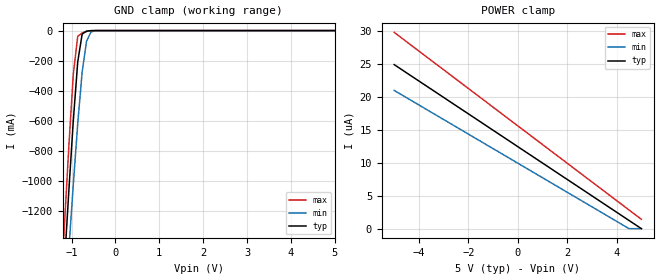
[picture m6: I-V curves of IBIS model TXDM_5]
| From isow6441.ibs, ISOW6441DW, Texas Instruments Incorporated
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|   TXDM_5 Model
[Model]   TXDM_5
Model_type Input
Polarity   Inverting
Enable   Active-High
Vinl =  1.500V
Vinh =  3.500V
C_comp   1.300pF   1.100pF   1.500pF
[Model Spec]
Vinh   3.500V   3.150V   3.850V
Vinl   1.500V   1.350V   1.650V
[Temperature Range]   27.000   0.150k   -55.000
[Voltage Range]   5.000V   4.500V   5.500V
[POWER Clamp Reference]   5.000V   4.500V   5.500V
[GND Clamp Reference]   0.0V   0.0V   0.0V
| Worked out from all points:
|   GND clamp passes 1 mA (typ) near -0.57 V on its own axis
[GND_clamp]
|Voltage   I(typ)   I(min)   I(max)
-5V       -17.32A    -16.15A    -18.32A
-1.263V   -2.058A    -2.361A    -1.839A
-1.162V   -1.554A    -1.904A    -1.294A
-1.061V   -1.063A    -1.456A    -767.3mA
-960mV    -599.4mA   -1.023A    -290.4mA
-859mV    -208mA     -619mA     -38.25mA
-758mV    -22.74mA   -275.5mA   -16.1mA
-657mV    -3.554mA   -69.14mA   -5.612mA
-556mV    -557.9uA   -9.055mA   -747.4uA
-455mV    -31.43uA   -673.6uA   -17.43uA
5V        0A         0A         0A
[POWER_clamp]
|Voltage   I(typ)   I(min)   I(max)
-5V       24.9uA     20.98uA    29.79uA
4.495V    1.257uA    11.35nA    2.851uA
4.596V    1.006uA    0A         2.565uA
5V        0A         0A         1.419uA
